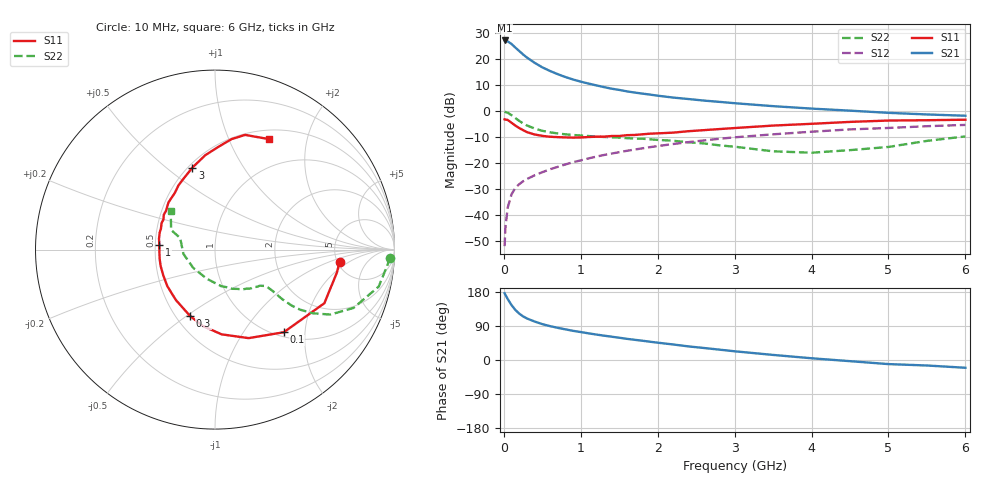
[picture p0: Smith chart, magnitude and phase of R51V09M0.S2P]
! SIEMENS Small Signal Semiconductors
! BFR183
! Si NPN RF Bipolar Junction Transistor in SOT23
! VCE = 1 V  IC = 9 mA
! Common Emitter S-Parameters:  May  1996
# GHz  S  MA  R  50
!  f  S11  S21  S12  S22
! GHz  MAG  ANG  MAG  ANG  MAG  ANG  MAG  ANG
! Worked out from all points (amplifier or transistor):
!   36 points, 10 MHz to 6 GHz, reference 50 ohm
!   highest |S21| = 27.3 dB at 10 MHz (marker M1)
!   |S21| within 3 dB of that: start of sweep to 159.5 MHz
!   unconditionally stable (mu >= 1): 732.6 MHz to 2.715 GHz
!   at 250 MHz: K = 0.61, MSG = 24.5 dB, |S12| = -27.0 dB
!   at 1.4 GHz: K = 1.07, MAG = 10.9 dB, |S12| = -16.3 dB
!   at 6 GHz: K = 0.93, MSG = 1.8 dB, |S12| = -5.3 dB
!   S11 on the Smith chart (normalised r, x): 10 MHz: 5.24, -1.36; 100 MHz: 1.08, -1.56; 300 MHz: 0.59, -0.52; 1 GHz: 0.53, +0.03; 3 GHz: 0.53, +0.62; 6 GHz: 0.61, +1.42
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0.01  0.6971 -5.5  23.13 176.2  0.0025 87.7  0.9763 -2.6
0.02  0.6912 -10.6  22.84 172.1  0.0056 86.3  0.9642 -5.2
0.05  0.6787 -26.1  22.16 161.0  0.0138 78.9  0.9353 -12.7
0.1  0.5991 -50.2  19.79 144.9  0.025 70.1  0.8381 -22.8
0.15  0.5276 -69.2  16.85 132.0  0.0333 63.0  0.7374 -29.4
0.2  0.4737 -85.5  14.48 122.5  0.0392 60.7  0.6516 -33.0
0.25  0.4314 -99.0  12.42 115.1  0.0445 58.7  0.5813 -35.2
0.3  0.3953 -110.5  10.84 109.6  0.0492 59.0  0.5313 -36.1
0.4  0.3555 -127.8  8.578 101.5  0.0582 59.2  0.464 -36.4
0.5  0.3349 -142.4  7.013 94.7  0.0666 60.2  0.4191 -35.9
0.6  0.322 -153.4  5.968 89.4  0.076 60.9  0.3911 -35.6
0.7  0.3164 -163.1  5.18 84.9  0.0845 61.8  0.373 -35.6
0.8  0.3124 -171.2  4.558 80.9  0.0941 61.8  0.3584 -35.6
1  0.3117 174.8  3.713 73.7  0.1128 62.0  0.3399 -36.5
1.1  0.3181 168.8  3.411 70.4  0.1229 62.0  0.332 -37.5
1.6  0.3452 145.7  2.414 55.8  0.1725 59.3  0.3023 -43.8
2.2  0.3862 125.6  1.833 41.0  0.2328 53.9  0.2696 -55.5
3  0.4736 105.5  1.427 23.0  0.3135 44.6  0.2067 -80.3
3.5  0.5286 95.9  1.252 13.4  0.3585 37.9  0.1686 -105.9
4.5  0.6223 81.5  1.025 -3.1  0.4459 24.9  0.1776 -172.3
5.5  0.6703 69.2  0.866 -14.5  0.514 13.1  0.2678 155.9
6  0.6856 63.9  0.818 -20.5  0.5443 5.4  0.3268 139.0
